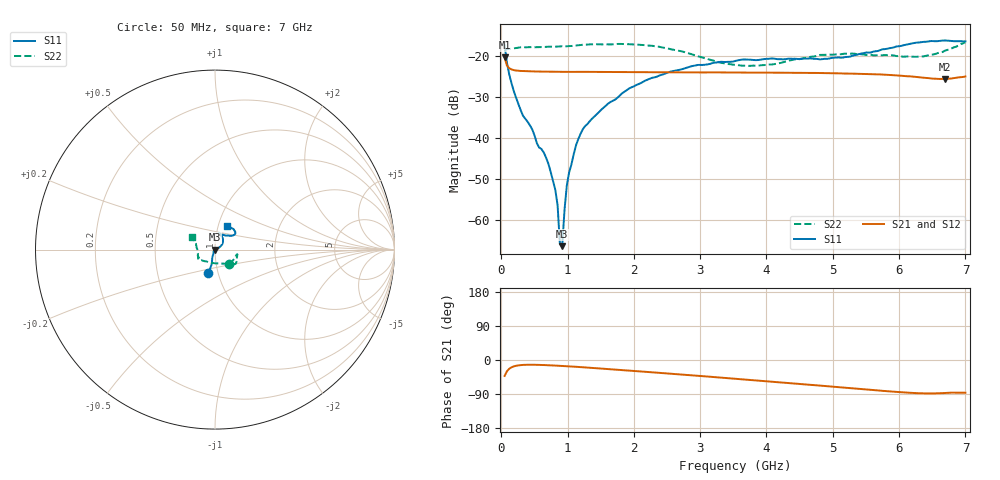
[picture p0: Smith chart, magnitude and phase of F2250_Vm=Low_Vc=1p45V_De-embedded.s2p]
! Integrated Device Technology
! Corporate Headquarters
! 6024 Silver Creek Valley Road
! San Jose, CA 95138  USA
! Phone:  1-408-284-8200
! Toll Free:  1-800-223-1366
! Webpage:  http://www.idt.com/
! Timing and RF Division
! 515 Groton Road, Suite 102
! Westford, MA 01886-6024
! Device:  F2250
! Description: Voltage Variable RF Attenuator
! Frequency:  50.0 -  6000.00 MHz
! Package:  3x3 mm Thin QFN Plastic Package: 16 pin
! Ports:  2 RF, 3 DC
!  Pin  1  = GND
!  Pin  2  = NC
!  Pin  3  = RF1  = Port 1
!  Pin  4  = NC
!  Pin  5  = GND
!  Pin  6  = GND
!  Pin  7  = GND
!  Pin  8  = GND
!  Pin  9  = NC
!  Pin 10  = RF2  = Port 2
!  Pin 11  = NC
!  Pin 12  = GND
!  Pin 13  = GND
!  Pin 14  = VCNTRL
!  Pin 15  = VDD
!  Pin 16  = VMODE
! Vcntrl:  1.450 Volts
! Vmode:  +0.000 Volts
! Vdd:  +3.30  Volts
! Current:  1.191 mA
! Data:  The device was measured on a the F2250 evaluation board which has
!  individual transmission lines to the RF pins.  Data was collected
!  using a calibrated network analyzer.  The evaluation board was
!  de-embedded using a TRL calibration technique.
!  The reference plane is the edge of the package pin.
! Misc:  SN 10
!  Action Tracker AT0258
! Date Measured:  2014-11-26
! Date:  2015-10-15  MJV
! Note:
!  Integrated Device Technology supplies this data as a sample of measured
!  data at the package pin for this product.  Your particular data for this
!  product may vary.
!  Data was taken at 25 degrees C.
!  Integrated Device Technology reserves the right to change this data at anytime.
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# GHz S dB R 50
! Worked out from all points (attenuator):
!   201 points, 50 MHz to 7 GHz, reference 50 ohm
!   highest |S21| = -20.38 dB at 50 MHz (marker M1); lowest = -25.6 dB at 6.687 GHz (marker M2)
!   lowest |S11| = -66.4 dB at 918.8 MHz (marker M3), VSWR 1.00, Z = 50 + j0.04 ohm
!   |S11| at or under -10 dB: start of sweep to end of sweep
!   |S22| runs from -22.4 to -16.7 dB; largest |S21 - S12| = 0.00025
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0.05  -17.30 -105.4  -20.38 -42.0  -20.37 -42.0  -18.90 -46.1
0.1195  -24.49 -105.4  -23.01 -23.1  -23.01 -23.1  -18.32 -17.3
0.22375  -30.23 -110.7  -23.58 -15.2  -23.57 -15.2  -18.09 -12.9
0.328  -34.61 -116.6  -23.70 -13.0  -23.70 -13.0  -17.90 -12.0
0.467  -37.92 -126.2  -23.79 -12.5  -23.80 -12.5  -17.89 -12.9
0.71025  -46.26 -131.6  -23.86 -13.8  -23.84 -13.8  -17.78 -17.7
0.8145  -52.63 -161.3  -23.87 -14.7  -23.86 -14.7  -17.75 -19.9
0.84925  -56.39 -159.3  -23.89 -15.1  -23.88 -15.1  -17.70 -20.6
0.884  -65.91 -155.0  -23.90 -15.4  -23.87 -15.4  -17.69 -21.4
0.91875  -66.36 56.2  -23.89 -15.7  -23.88 -15.7  -17.68 -22.2
0.9535  -57.54 -57.8  -23.90 -16.1  -23.88 -16.1  -17.76 -22.7
0.98825  -51.59 -18.3  -23.91 -16.4  -23.89 -16.4  -17.67 -23.1
1.023  -48.39 -6.8  -23.91 -16.8  -23.88 -16.8  -17.62 -23.3
1.12725  -41.77 10.5  -23.89 -17.9  -23.89 -17.9  -17.46 -25.1
1.2315  -37.81 15.4  -23.89 -19.1  -23.89 -19.2  -17.29 -27.1
1.857  -28.73 30.6  -23.96 -27.1  -23.93 -27.1  -17.11 -34.2
2.37825  -24.84 40.8  -23.99 -33.8  -24.00 -33.8  -17.78 -39.7
3.525  -21.26 69.5  -24.07 -49.3  -24.06 -49.3  -22.19 -84.2
4.7065  -20.71 70.8  -24.18 -66.0  -24.18 -66.0  -20.16 -142.3
5.85325  -18.14 38.8  -24.65 -82.8  -24.67 -82.8  -19.90 -160.3
6.68725  -16.25 47.9  -25.64 -87.1  -25.63 -87.1  -18.77 160.0
7  -16.46 62.7  -25.03 -86.4  -25.02 -86.5  -16.67 152.3
